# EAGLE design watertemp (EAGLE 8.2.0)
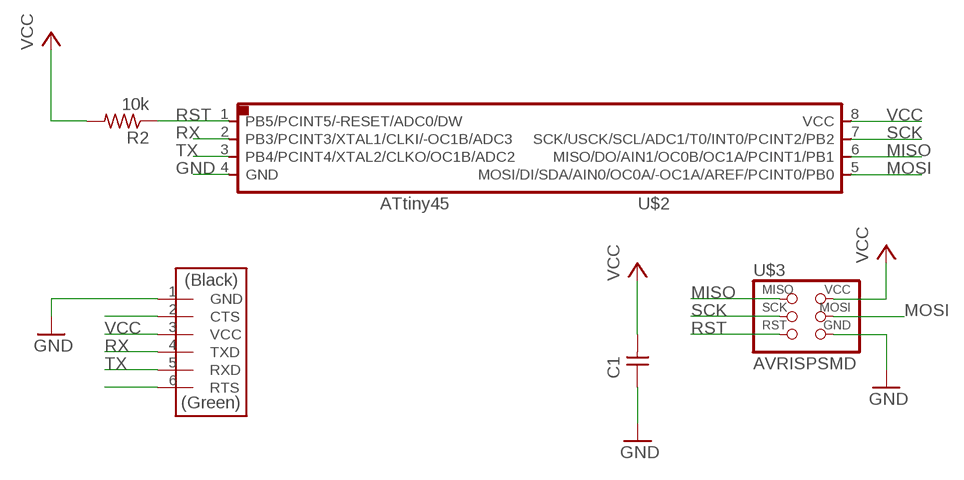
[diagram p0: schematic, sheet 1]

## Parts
C1  CAP-UNPOLARIZEDFAB  [C1206FAB]
R2  10k  RES-US1206FAB  [R1206FAB]
U$2  ATTINY45SI  [SOIC8]
U$3  AVRISPSMD  [2X03SMD]
U$4  FTDI-SMD-HEADER  [1X06SMD]

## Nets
GND: C1.1 U$2.4(GND) U$3.6(GND) U$4.1(GND)
MISO: U$2.6(MISO/DO/AIN1/OC0B/OC1A/PCINT1/PB1) U$3.1(MISO)
MOSI: U$2.5(MOSI/DI/SDA/AIN0/OC0A/-OC1A/AREF/PCINT0/PB0) U$3.4(MOSI)
N$10: U$4.2(CTS)
N$14: U$4.6(RTS)
RST: R2.1 U$2.1(PB5/PCINT5/-RESET/ADC0/DW) U$3.5(RST)
RX: U$2.2(PB3/PCINT3/XTAL1/CLKI/-OC1B/ADC3) U$4.4(TXD)
SCK: U$2.7(SCK/USCK/SCL/ADC1/T0/INT0/PCINT2/PB2) U$3.3(SCK)
TX: U$2.3(PB4/PCINT4/XTAL2/CLKO/OC1B/ADC2) U$4.5(RXD)
VCC: C1.2 R2.2 U$2.8(VCC) U$3.2(VCC) U$4.3(VCC)

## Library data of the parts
C1 = fab:CAP-UNPOLARIZED
R2 = fab:RES-US: Resistor (US Symbol)
U$2 = fab:ATTINY45
U$3 = fab:AVRISP
U$4 = fab:FTDI-SMD-HEADER

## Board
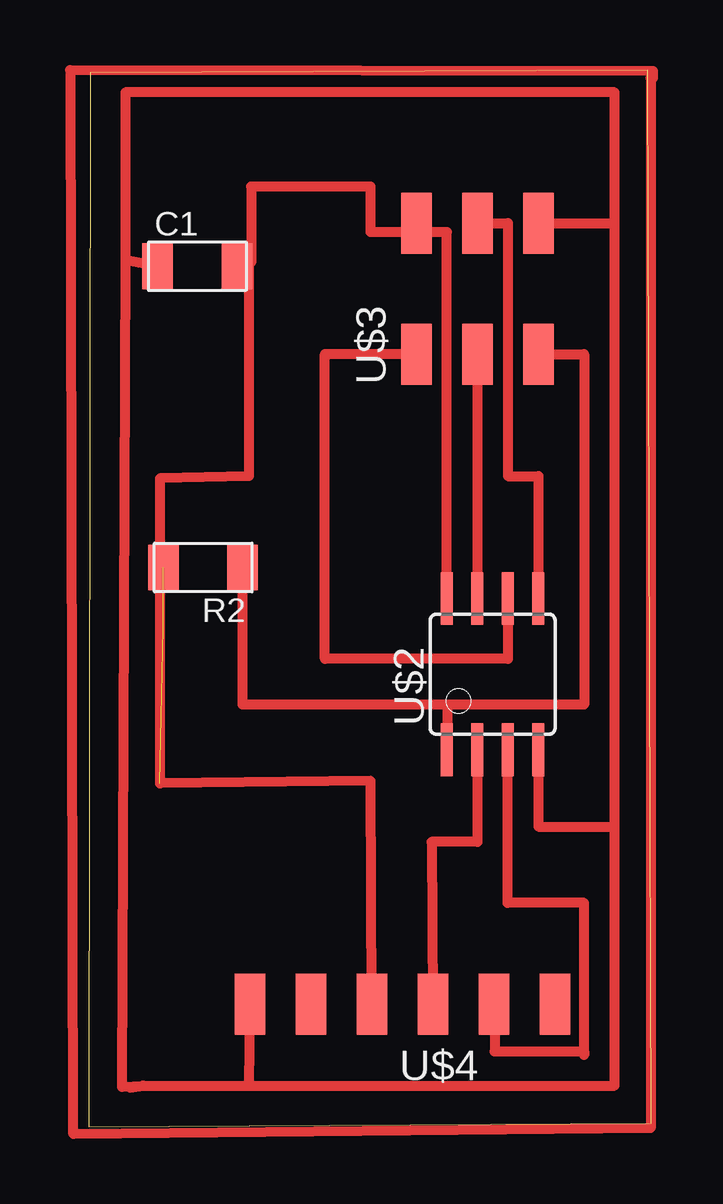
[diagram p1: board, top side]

Size 23.42 x 44.02 mm. Coordinates in mm from the lower left corner, seen from the top.
Outline: 0,0 23.42,0.15 23.27,44.02 0.05,43.92 0,0
Copper layers (1*16): Top 0.035mm / dielectric 1.5mm / Bottom 0.035mm
Design rules "default *": minimum track width 16mil, minimum drill 24mil, track to track 12mil, track to pad 12mil, pad to pad 12mil, via to via 8mil, smd to smd 8mil, copper to edge 40mil, drill to drill 8mil, minimum pad ring 10mil, minimum via ring 8mil, stop-mask expansion 4mil, vias tented up to drill 0mil, thermal gap 10mil

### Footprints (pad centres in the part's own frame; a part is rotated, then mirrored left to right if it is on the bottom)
C1206FAB = smd 1.27 x 1.905: 1 -1.651,0; 2 1.651,0
R1206FAB = smd 1.27 x 1.905: 1 -1.651,0; 2 1.651,0
SOIC8 = smd 0.5 x 2.2: 1 -1.905,-3.154; 2 -0.645,-3.154; 3 0.625,-3.154; 4 1.895,-3.154; 5 1.905,3.154; 6 0.635,3.154; 7 -0.635,3.154; 8 -1.905,3.154
2X03SMD = smd 2.54 x 1.27: 1 -2.54,2.54; 2 2.92,2.54; 3 -2.54,0; 4 2.92,0; 5 -2.54,-2.54; 6 2.92,-2.54
1X06SMD = smd 2.54 x 1.27: 1 0,6.35; 2 0,3.81; 3 0,1.27; 4 0,-1.27; 5 0,-3.81; 6 0,-6.35

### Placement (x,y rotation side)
C1  4.52,35.86 0 top
R2  4.76,23.31 180 top
U$2  16.82,18.86 0 top
U$3  16.19,34.74 90 top
U$4  13.06,5.12 90 top

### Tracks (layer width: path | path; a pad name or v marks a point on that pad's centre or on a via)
GND
  Top 0.406: 1.71,1.63 2.26,1.72 | 2.26,1.72 6.66,1.72 | 6.66,1.72 21.9,1.72 21.9,12.51 | 21.9,12.51 21.9,37.66 | 21.9,37.66 21.9,43.11 1.52,43.11 1.52,36.11 | 1.52,36.11 1.37,1.67 2.26,1.72 | C1.1 1.52,36.11 | U$4.1 6.66,1.72 | U$2.4 18.73,12.51 21.9,12.51 | U$3.6 21.9,37.66
MISO
  Top 0.406: 9.83,32.2 9.94,32.16 | U$3.1 9.83,32.2 | U$2.6 17.45,19.5 9.83,19.5 9.83,32.2
MOSI
  Top 0.406: U$2.5 18.73,27.12 17.45,27.12 17.45,37.66 U$3.4 16.59,37.69 16.52,37.69 16.37,38.1 16.51,37.8
N$2
  Top 0.406: -0.8,44.05 23.5,44 23.5,43.7 23.4,43.7 23.4,-0.05 -0.65,-0.3 -0.75,43.9
RST
  Top 0.406: U$3.5 20.63,32.2 20.63,17.59 14.95,17.59 | 14.95,17.59 6.41,17.59 R2.1 | U$2.1 14.95,15.71 14.95,17.59
RX
  Top 0.406: U$2.2 16.19,11.88 14.28,11.88 U$4.4
SCK
  Top 0.406: U$3.3 U$2.7
TX
  Top 0.406: U$2.3 17.45,9.34 20.63,9.34 20.63,3.15 | U$4.5 16.9,6.17 16.9,3.15 20.63,3.15 | 20.63,3.15 20.63,2.99
VCC  (2 unrouted)
  Top 0.406: C1.2 6.66,36.01 | 6.66,36.01 6.76,36.01 6.76,39.19 11.74,39.19 11.74,37.28 13.65,37.28 | 6.66,36.01 6.66,27.12 2.95,27.02 2.95,14.32 11.74,14.42 U$4.3 | U$2.8 14.92,37.28 13.65,37.28 | 13.65,37.28 U$3.2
